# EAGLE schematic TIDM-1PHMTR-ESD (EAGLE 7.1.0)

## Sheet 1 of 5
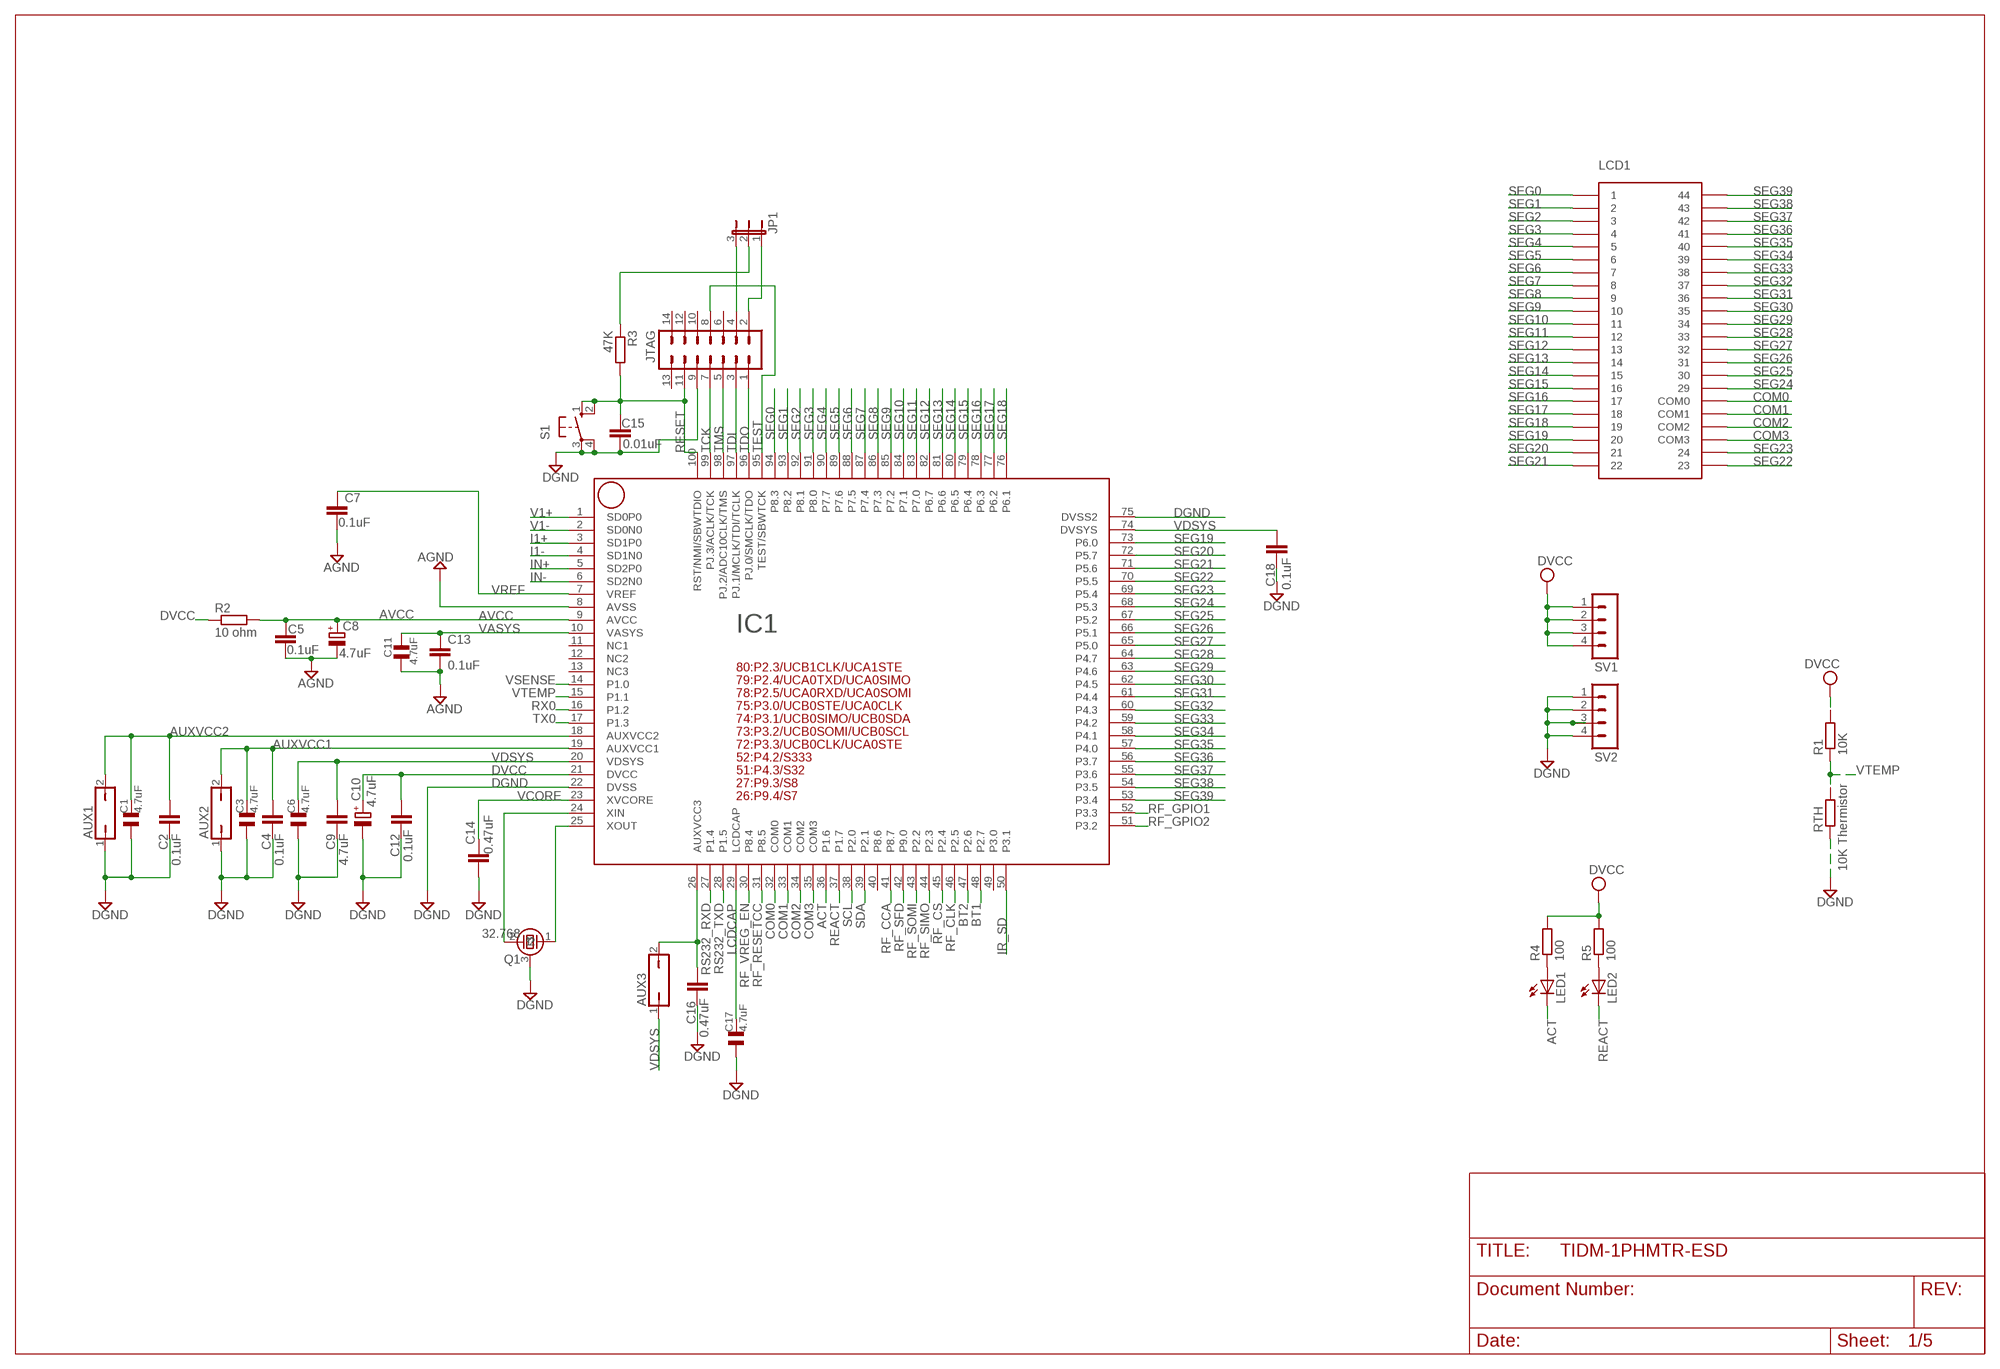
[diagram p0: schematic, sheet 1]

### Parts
AUX1  JP1Q  [JP1]
AUX2  JP1Q  [JP1]
AUX3  JP1Q  [JP1]
C1  4.7uF  C_0805  [0805]
C2  0.1uF  C-EUC0603  [C0603]
C3  4.7uF  C_0805  [0805]
C4  0.1uF  C-EUC0603  [C0603]
C5  0.1uF  C-EUC0603  [C0603]
C6  4.7uF  C_0805  [0805]
C7  0.1uF  C-EUC0603  [C0603]
C8  4.7uF  CPOL-EUSMCB  [SMC_B]
C9  4.7uF  C-EUC0603  [C0603]
C10  4.7uF  CPOL-EUSMCB  [SMC_B]
C11  4.7uF  C_0805  [0805]
C12  0.1uF  C-EUC0603  [C0603]
C13  0.1uF  C-EUC0603  [C0603]
C14  0.47uF  C-EUC0603  [C0603]
C15  0.01uF  C-EUC0603  [C0603]
C16  0.47uF  C-EUC0603  [C0603]
C17  4.7uF  C_0805  [0805]
C18  0.1uF  C-EUC0603  [C0603]
IC1  F6733---PZ100  [PZ100]
JP1  JP2E  [JP2]
JTAG  MA07-2MA07-2JTAG  [MA07-2JTAG]
LCD1  TI_160SEG_LCD  [TI_160SEG_LCD]
LED1  LED3MM  [LED3MM]
LED2  LED3MM  [LED3MM]
Q1  32.768  CRYSTAL-LSDTC26H-1  [TC26H-1]
R1  10K  R-EU_R0603  [R0603]
R2  10 ohm  R-EU_R0603  [R0603]
R3  47K  R-EU_R0603  [R0603]
R4  100  R-EU_R0603  [R0603]
R5  100  R-EU_R0603  [R0603]
RTH  10K Thermistor  R-EU_R0603  [R0603]
S1  10-XX  [B3F-10XX]
SV1  MA04-1  [MA04-1]
SV2  MA04-1  [MA04-1]

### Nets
ACT: IC1.36(P1.6) LED1.K(C) ; also sheet 4
AGND: C5.2 C7.2 C8.- C11.1 C13.2 IC1.8(AVSS) ; also sheet 2
AUXVCC1: AUX2.2 C3.2 C4.2 IC1.19(AUXVCC1)
AUXVCC2: AUX1.2 C1.2 C2.2 IC1.18(AUXVCC2)
AVCC: C5.1 C8.+ IC1.9(AVCC) R2.2 ; also sheet 2
BT1: IC1.48(P2.7) ; also sheet 4
BT2: IC1.47(P2.6) ; also sheet 4
COM0: IC1.32(COM0) LCD1.COM0
COM1: IC1.33(COM1) LCD1.COM1
COM2: IC1.34(COM2) LCD1.COM2
COM3: IC1.35(COM3) LCD1.COM3
DGND: AUX1.1 AUX2.1 C1.1 C2.1 C3.1 C4.1 C6.1 C9.1 C10.- C12.1 C14.1 C15.2 C16.1 C17.1 C18.1 IC1.22(DVSS) IC1.75(DVSS2) JTAG.9 Q1.3 RTH.1 S1.3(P) S1.4(P1) SV2.1 SV2.2 SV2.3 SV2.4 ; also sheet 3,4,5
DVCC: C10.+ C12.2 IC1.21(DVCC) JP1.2 R1.2 R2.1 R3.1 R4.2 R5.2 SV1.1 SV1.2 SV1.3 SV1.4 ; also sheet 3,4,5
I1+: IC1.3(SD1P0) ; also sheet 2
I1-: IC1.4(SD1N0) ; also sheet 2
IN+: IC1.5(SD2P0) ; also sheet 2
IN-: IC1.6(SD2N0) ; also sheet 2
IR_SD: IC1.50(P3.1) ; also sheet 4
JTAG_EXT: JP1.3 JTAG.4
JTAG_INT: JP1.1 JTAG.2
LCDCAP: C17.2 IC1.29(LCDCAP)
N$38: AUX3.2 C16.2 IC1.26(AUXVCC3)
N$104: LED1.A R4.1
N$105: LED2.A R5.1
REACT: IC1.37(P1.7) LED2.K(C) ; also sheet 4
RESET: C15.1 IC1.100(RST/NMI/SBWTDIO) JTAG.11 R3.2 S1.1(S) S1.2(S1)
RF_CCA: IC1.41(P8.7) ; also sheet 4
RF_CLK: IC1.46(P2.5) ; also sheet 4
RF_CS: IC1.45(P2.4) ; also sheet 4
RF_GPIO1: IC1.52(P3.3) ; also sheet 4
RF_GPIO2: IC1.51(P3.2) ; also sheet 4
RF_RESETCC: IC1.31(P8.5) ; also sheet 4
RF_SFD: IC1.42(P9.0) ; also sheet 4
RF_SIMO: IC1.44(P2.3) ; also sheet 4
RF_SOMI: IC1.43(P2.2) ; also sheet 4
RF_VREG_EN: IC1.30(P8.4) ; also sheet 4
RS232_RXD: IC1.27(P1.4) ; also sheet 5
RS232_TXD: IC1.28(P1.5) ; also sheet 5
RX0: IC1.16(P1.2) ; also sheet 4
SCL: IC1.38(P2.0) ; also sheet 4
SDA: IC1.39(P2.1) ; also sheet 4
SEG0: IC1.94(P8.3) LCD1.1
SEG1: IC1.93(P8.2) LCD1.2
SEG2: IC1.92(P8.1) LCD1.3
SEG3: IC1.91(P8.0) LCD1.4
SEG4: IC1.90(P7.7) LCD1.5
SEG5: IC1.89(P7.6) LCD1.6
SEG6: IC1.88(P7.5) LCD1.7
SEG7: IC1.87(P7.4) LCD1.8
SEG8: IC1.86(P7.3) LCD1.9
SEG9: IC1.85(P7.2) LCD1.10
SEG10: IC1.84(P7.1) LCD1.11
SEG11: IC1.83(P7.0) LCD1.12
SEG12: IC1.82(P6.7) LCD1.13
SEG13: IC1.81(P6.6) LCD1.14
SEG14: IC1.80(P6.5) LCD1.15
SEG15: IC1.79(P6.4) LCD1.16
SEG16: IC1.78(P6.3) LCD1.17
SEG17: IC1.77(P6.2) LCD1.18
SEG18: IC1.76(P6.1) LCD1.19
SEG19: IC1.73(P6.0) LCD1.20
SEG20: IC1.72(P5.7) LCD1.21
SEG21: IC1.71(P5.6) LCD1.22
SEG22: IC1.70(P5.5) LCD1.23
SEG23: IC1.69(P5.4) LCD1.24
SEG24: IC1.68(P5.3) LCD1.29
SEG25: IC1.67(P5.2) LCD1.30
SEG26: IC1.66(P5.1) LCD1.31
SEG27: IC1.65(P5.0) LCD1.32
SEG28: IC1.64(P4.7) LCD1.33
SEG29: IC1.63(P4.6) LCD1.34
SEG30: IC1.62(P4.5) LCD1.35
SEG31: IC1.61(P4.4) LCD1.36
SEG32: IC1.60(P4.3) LCD1.37
SEG33: IC1.59(P4.2) LCD1.38
SEG34: IC1.58(P4.1) LCD1.39
SEG35: IC1.57(P4.0) LCD1.40
SEG36: IC1.56(P3.7) LCD1.41
SEG37: IC1.55(P3.6) LCD1.42
SEG38: IC1.54(P3.5) LCD1.43
SEG39: IC1.53(P3.4) LCD1.44
TCK: IC1.99(PJ.3/ACLK/TCK) JTAG.7
TDI: IC1.97(PJ.1/MCLK/TDI/TCLK) JTAG.3
TDO: IC1.96(PJ.0/SMCLK/TDO) JTAG.1
TEST: IC1.95(TEST/SBWTCK) JTAG.8
TMS: IC1.98(PJ.2/ADC10CLK/TMS) JTAG.5
TX0: IC1.17(P1.3) ; also sheet 4
V1+: IC1.1(SD0P0) ; also sheet 2
V1-: IC1.2(SD0N0) ; also sheet 2
VASYS: C11.2 C13.1 IC1.10(VASYS)
VCORE: C14.2 IC1.23(XVCORE)
VDSYS: AUX3.1 C6.2 C9.2 C18.2 IC1.20(VDSYS) IC1.74(DVSYS)
VREF: C7.1 IC1.7(VREF)
VSENSE: IC1.14(P1.0) ; also sheet 3
VTEMP: IC1.15(P1.1) R1.1 RTH.2
XIN1: IC1.24(XIN) Q1.2
XOUT1: IC1.25(XOUT) Q1.1
Unconnected: IC1.11(NC1) IC1.12(NC2) IC1.13(NC3) IC1.40(P8.6) IC1.49(P3.0) JTAG.6 JTAG.10 JTAG.12 JTAG.13 JTAG.14

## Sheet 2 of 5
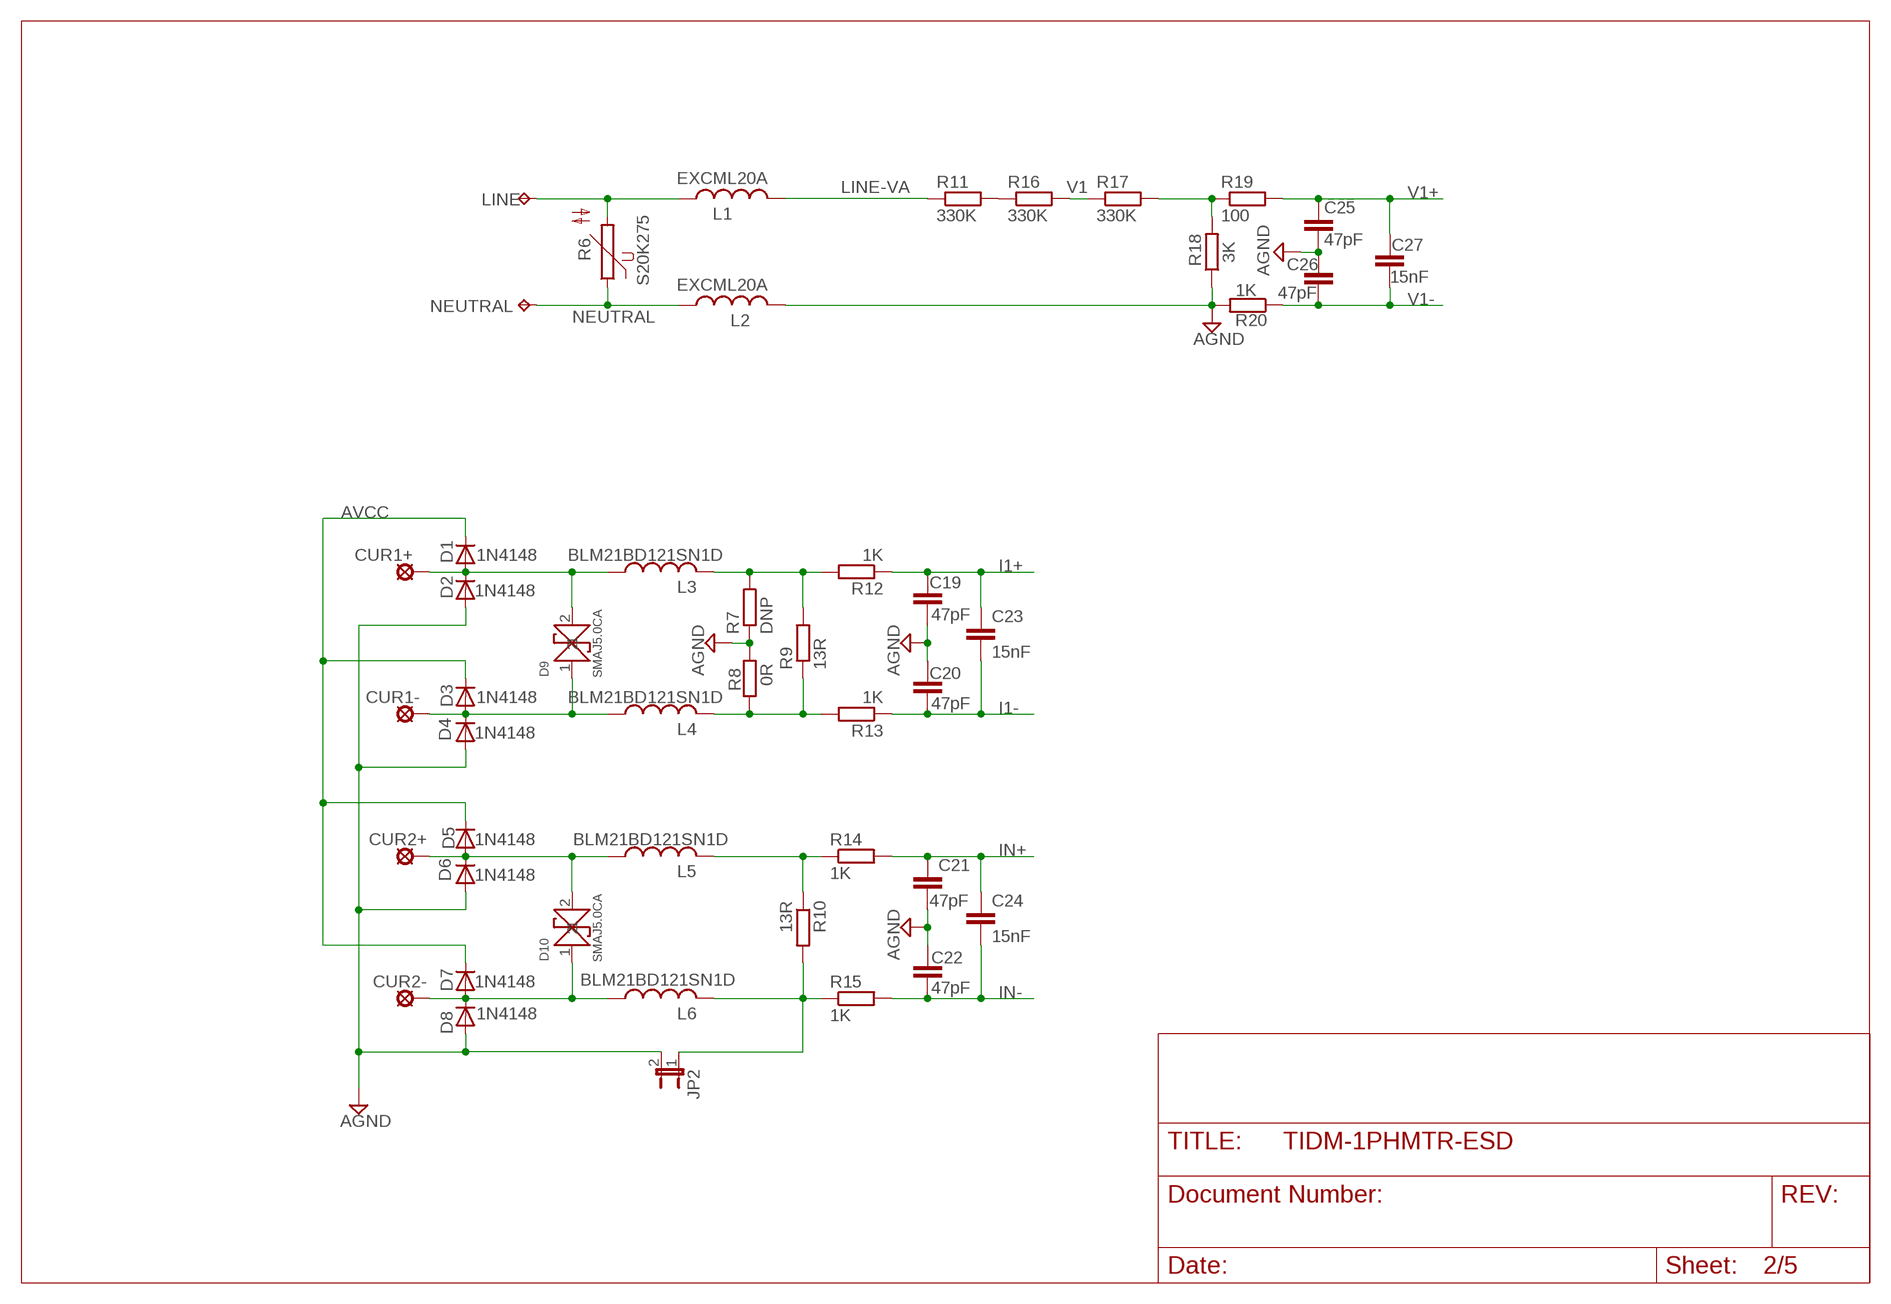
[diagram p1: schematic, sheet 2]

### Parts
C19  47pF  C-EUC0603  [C0603]
C20  47pF  C-EUC0603  [C0603]
C21  47pF  C-EUC0603  [C0603]
C22  47pF  C-EUC0603  [C0603]
C23  15nF  C-EUC0603  [C0603]
C24  15nF  C-EUC0603  [C0603]
C25  47pF  C-EUC0603  [C0603]
C26  47pF  C-EUC0603  [C0603]
C27  15nF  C-EUC0603  [C0603]
CUR1+  LSP10  [LSP10]
CUR1-  LSP10  [LSP10]
CUR2+  LSP10  [LSP10]
CUR2-  LSP10  [LSP10]
D1  1N4148  1N4148SOD80C  [SOD80C]
D2  1N4148  1N4148SOD80C  [SOD80C]
D3  1N4148  1N4148SOD80C  [SOD80C]
D4  1N4148  1N4148SOD80C  [SOD80C]
D5  1N4148  1N4148SOD80C  [SOD80C]
D6  1N4148  1N4148SOD80C  [SOD80C]
D7  1N4148  1N4148SOD80C  [SOD80C]
D8  1N4148  1N4148SOD80C  [SOD80C]
D9  SMAJ5.0CA  SMAJ  [DO-214]
D10  SMAJ5.0CA  SMAJ  [DO-214]
JP2  JP1E  [JP1]
L1  EXCML20A  L-US08050805  [0805@1]
L2  EXCML20A  L-US08050805  [0805@1]
L3  BLM21BD121SN1D  L-USL2012C  [L2012C]
L4  BLM21BD121SN1D  L-USL2012C  [L2012C]
L5  BLM21BD121SN1D  L-USL2012C  [L2012C]
L6  BLM21BD121SN1D  L-USL2012C  [L2012C]
LINE  TPPAD1-20  [P1-20]
NEUTRAL  TPPAD1-20  [P1-20]
R6  S20K275  S20K680S20K680-1  [S20K680-1]
R7  DNP  R-EU_R0603  [R0603]
R8  0R  R-EU_R0603  [R0603]
R9  13R  R-EU_R0603  [R0603]
R10  13R  R-EU_R0603  [R0603]
R11  330K  R-EU_R0603  [R0603]
R12  1K  R-EU_R0603  [R0603]
R13  1K  R-EU_R0603  [R0603]
R14  1K  R-EU_R0603  [R0603]
R15  1K  R-EU_R0603  [R0603]
R16  330K  R-EU_R0603  [R0603]
R17  330K  R-EU_R0603  [R0603]
R18  3K  R-EU_R0603  [R0603]
R19  100  R-EU_R0603  [R0603]
R20  1K  R-EU_R0603  [R0603]

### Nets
AGND: C19.2 C20.1 C21.2 C22.1 C25.2 C26.1 D2.A D4.A D6.A D8.A JP2.2 L2.2 R7.1 R8.2 R18.1 R20.2 ; also sheet 1
AVCC: D1.C D3.C D5.C D7.C ; also sheet 1
I1+: C19.1 C23.1 R12.1 ; also sheet 1
I1-: C20.2 C23.2 R13.1 ; also sheet 1
IN+: C21.1 C24.1 R14.2 ; also sheet 1
IN-: C22.2 C24.2 R15.2 ; also sheet 1
LINE-VA: L1.2 R11.1 ; also sheet 3
N$5: L1.1 LINE.TP R6.2
N$19: CUR1+.MP D1.A D2.C D9.2 L3.1
N$20: CUR1-.MP D3.A D4.C D9.1 L4.1
N$21: CUR2+.MP D5.A D6.C D10.2 L5.1
N$22: CUR2-.MP D7.A D8.C D10.1 L6.1
N$24: JP2.1 L6.2 R10.2 R15.1
N$27: L4.2 R8.1 R9.1 R13.2
N$31: L5.2 R10.1 R14.1
N$32: R17.2 R18.2 R19.1
N$39: R11.2 R16.1
N$42: L3.2 R7.2 R9.2 R12.2
NEUTRAL: L2.1 NEUTRAL.TP R6.1 ; also sheet 3
V1: R16.2 R17.1
V1+: C25.1 C27.1 R19.2 ; also sheet 1
V1-: C26.2 C27.2 R20.1 ; also sheet 1

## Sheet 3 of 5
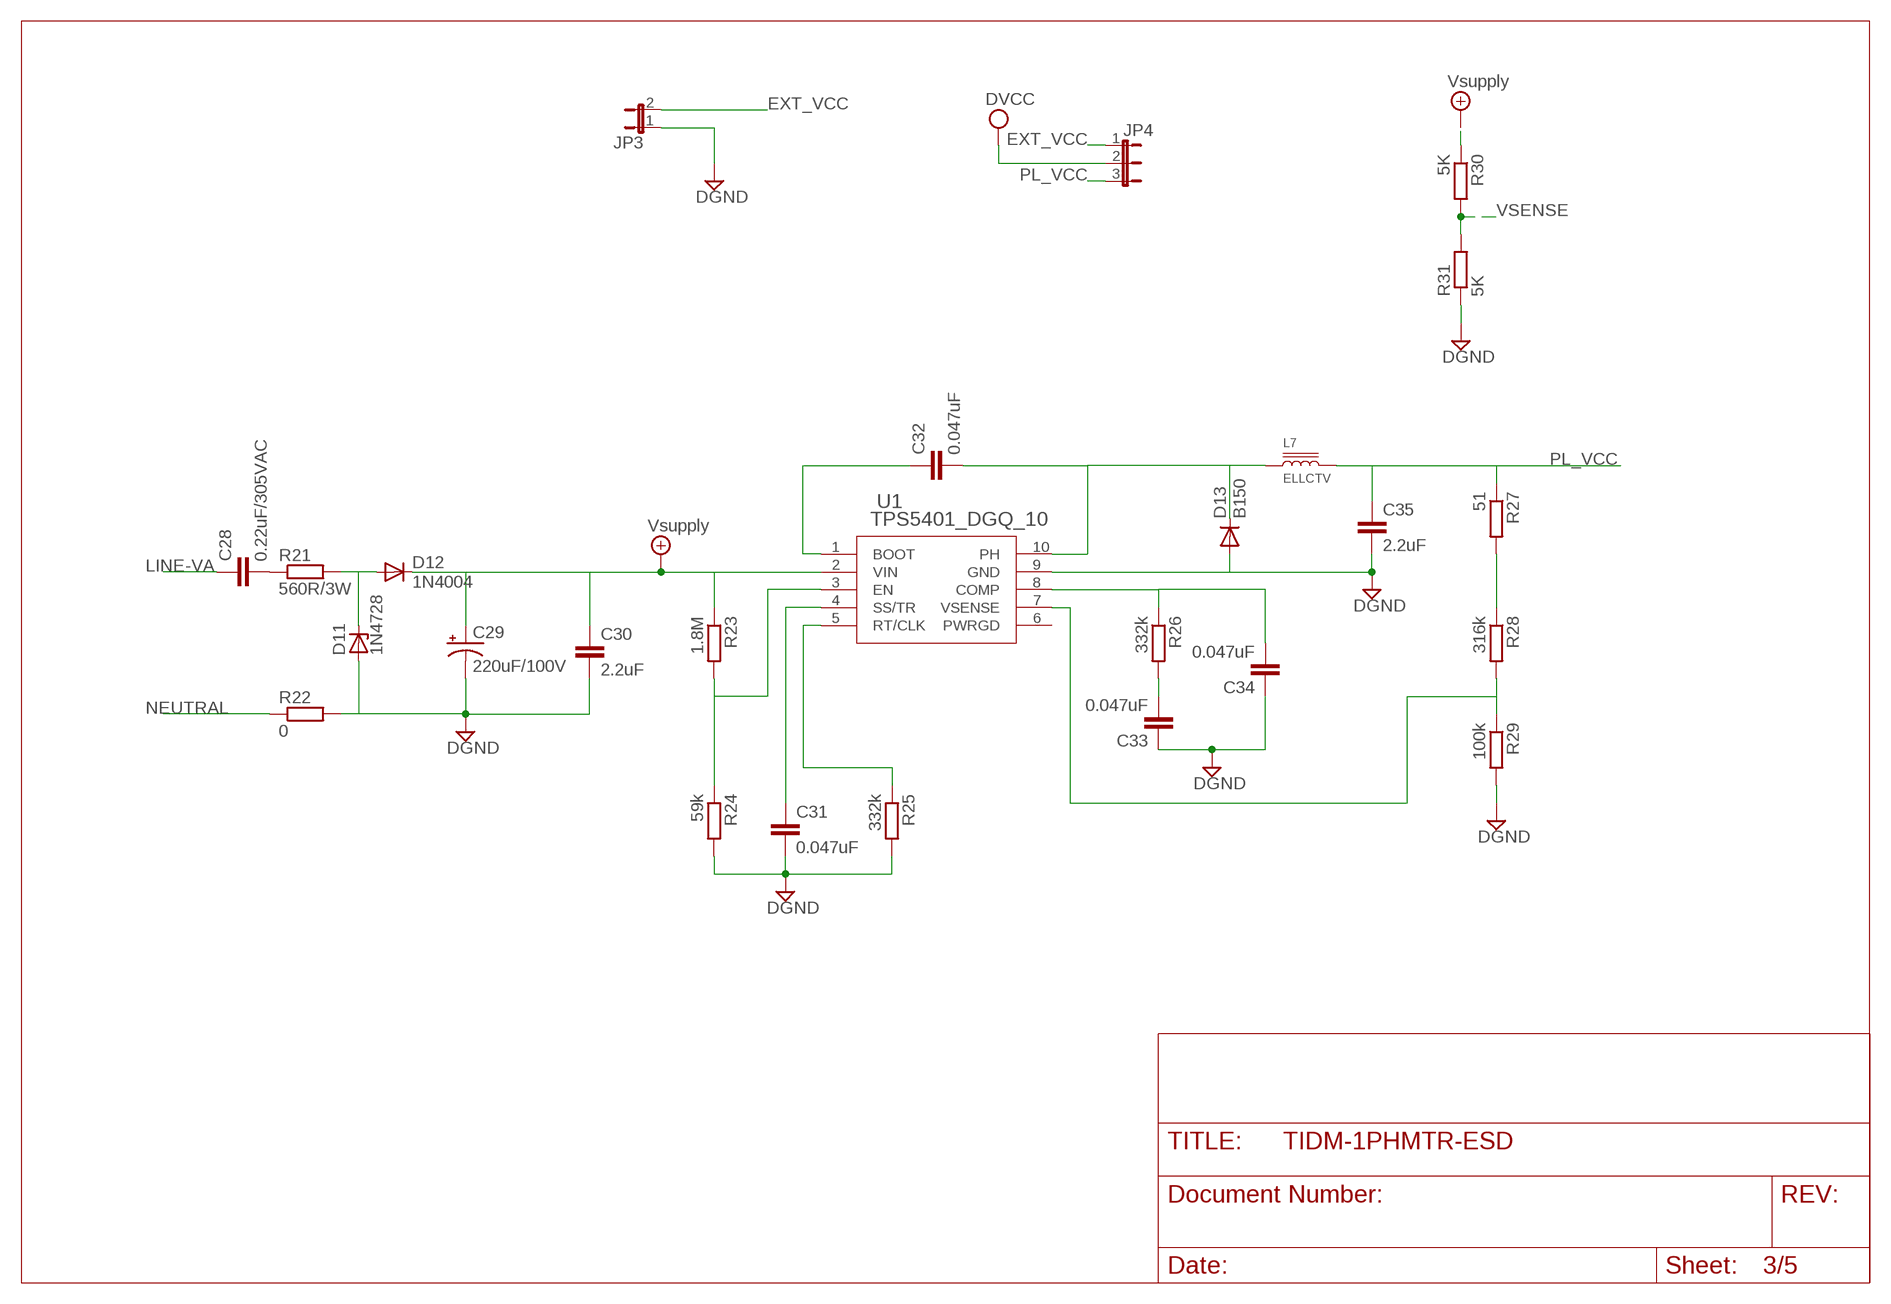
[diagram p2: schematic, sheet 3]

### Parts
C28  0.22uF/305VAC  C15/8  [C15B8]
C29  220uF/100V  CPOL-USE5-13  [E5-13]
C30  2.2uF  C-EUC1206  [C1206]
C31  0.047uF  C-EUC0603  [C0603]
C32  0.047uF  C-EUC0603  [C0603]
C33  0.047uF  C-EUC0603  [C0603]
C34  0.047uF  C-EUC0603  [C0603]
C35  2.2uF  C-EUC1206  [C1206]
D11  1N4728  [DO41Z10]
D12  1N4004  [DO41-10]
D13  B150  DIODE-DO214BA  [DO214BA]
JP3  JP1E  [JP1]
JP4  JP2E  [JP2]
L7  ELLCTV  [ELLCTV]
R21  560R/3W  R-EU_0414/15  [0414/15]
R22  0  R-EU_R0805  [R0805]
R23  1.8M  R-EU_R0603  [R0603]
R24  59k  R-EU_R0603  [R0603]
R25  332k  R-EU_R0603  [R0603]
R26  332k  R-EU_R0603  [R0603]
R27  51  R-EU_R0603  [R0603]
R28  316k  R-EU_R0603  [R0603]
R29  100k  R-EU_R0603  [R0603]
R30  5K  R-EU_R0603  [R0603]
R31  5K  R-EU_R0603  [R0603]
U1  TPS5401_DGQ_10  [DGQ10_1P88X1P57]

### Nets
+9V: C29.+ C30.1 D12.C R23.1 R30.1 U1.2(VIN) ; supply symbol labelled Vsupply
DGND: C29.- C30.2 C31.2 C33.1 C34.1 C35.2 D11.A D13.A JP3.1 R22.2 R24.2 R25.2 R29.2 R31.1 U1.9(GND) ; also sheet 1,4,5
DVCC: JP4.2 ; also sheet 1,4,5
EXT_VCC: JP3.2 JP4.1
LINE-VA: C28.1 ; also sheet 2
N$1: C28.2 R21.1
N$3: D11.C D12.A R21.2
N$7: R23.2 R24.1 U1.3(EN)
N$12: C31.1 U1.4(SS/TR)
N$13: R25.1 U1.5(RT/CLK)
N$23: C33.2 R26.2
N$25: R27.2 R28.1
N$26: C34.2 R26.1 U1.8(COMP)
N$28: C32.1 U1.1(BOOT)
N$29: C32.2 D13.C L7.1 U1.10(PH)
N$34: R28.2 R29.1 U1.7(VSENSE)
NEUTRAL: R22.1 ; also sheet 2
PL_VCC: C35.1 JP4.3 L7.2 R27.1
VSENSE: R30.2 R31.2 ; also sheet 1
Unconnected: U1.6(PWRGD)

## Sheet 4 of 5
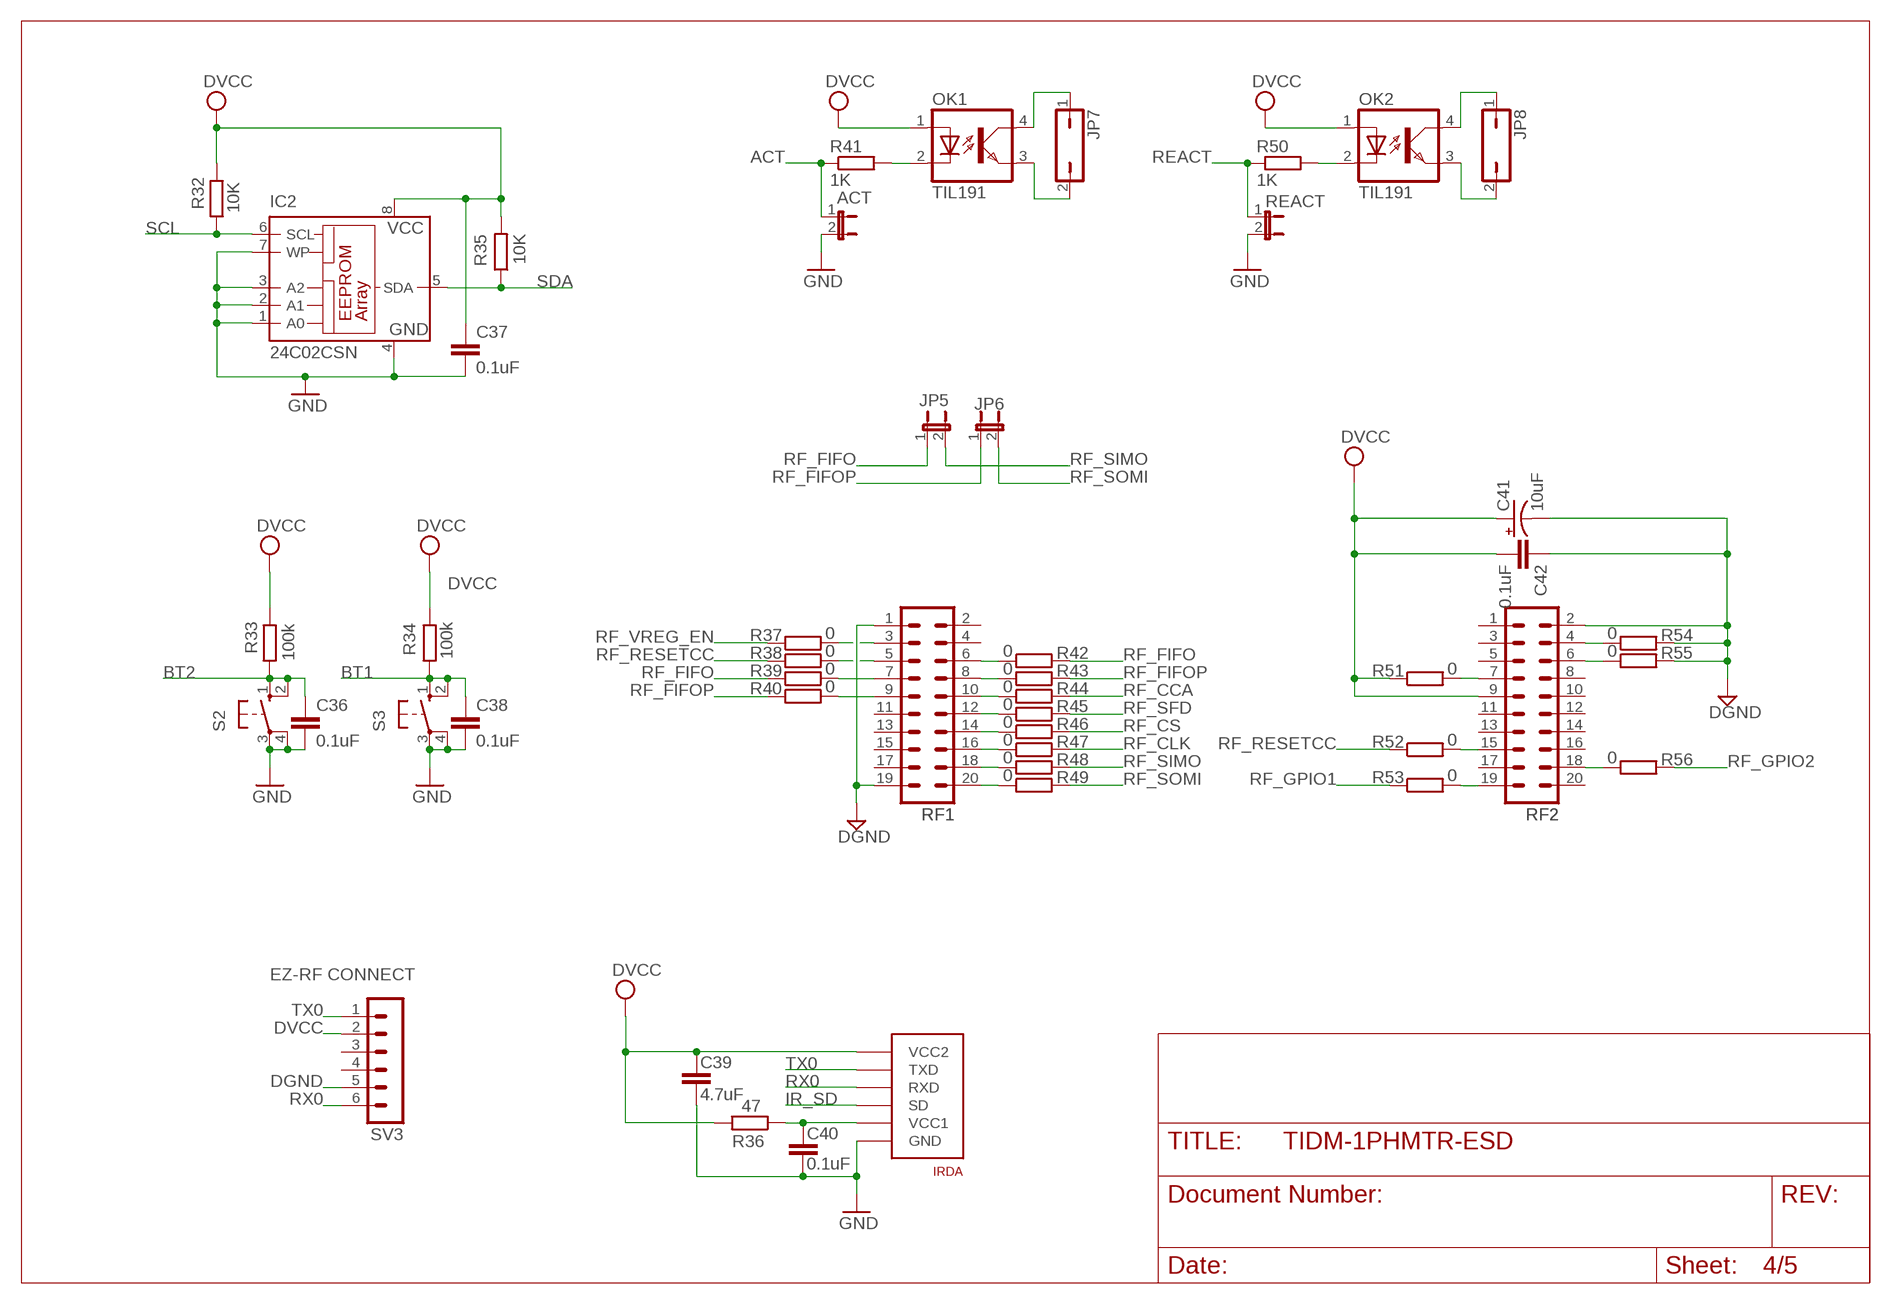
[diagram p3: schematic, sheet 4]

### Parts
ACT  JP1E  [JP1]
C36  0.1uF  C-EUC0603  [C0603]
C37  0.1uF  C-EUC0603  [C0603]
C38  0.1uF  C-EUC0603  [C0603]
C39  4.7uF  C-EUC0603  [C0603]
C40  0.1uF  C-EUC0603  [C0603]
C41  10uF  CPOL-USCT3216  [CT3216]
C42  0.1uF  C-EUC0603  [C0603]
IC2  24C02CSN  [SO-08]
IRDA  TFBS4711-TT1  [TFBS4711]
JP5  JP1E  [JP1]
JP6  JP1E  [JP1]
JP7  JP1Q  [JP1]
JP8  JP1Q  [JP1]
OK1  TIL191  [DIL04]
OK2  TIL191  [DIL04]
R32  10K  R-EU_R0603  [R0603]
R33  100k  R-EU_R0603  [R0603]
R34  100k  R-EU_R0603  [R0603]
R35  10K  R-EU_R0603  [R0603]
R36  47  R-EU_R0603  [R0603]
R37  0  R-EU_R0603  [R0603]
R38  0  R-EU_R0603  [R0603]
R39  0  R-EU_R0603  [R0603]
R40  0  R-EU_R0603  [R0603]
R41  1K  R-EU_R0603  [R0603]
R42  0  R-EU_R0603  [R0603]
R43  0  R-EU_R0603  [R0603]
R44  0  R-EU_R0603  [R0603]
R45  0  R-EU_R0603  [R0603]
R46  0  R-EU_R0603  [R0603]
R47  0  R-EU_R0603  [R0603]
R48  0  R-EU_R0603  [R0603]
R49  0  R-EU_R0603  [R0603]
R50  1K  R-EU_R0603  [R0603]
R51  0  R-EU_R0603  [R0603]
R52  0  R-EU_R0603  [R0603]
R53  0  R-EU_R0603  [R0603]
R54  0  R-EU_R0603  [R0603]
R55  0  R-EU_R0603  [R0603]
R56  0  R-EU_R0603  [R0603]
REACT  JP1E  [JP1]
RF1  TFM-110-02-SM-D-A-K  [TFM-110-02-SM-D-A-K]
RF2  TFM-110-02-SM-D-A-K  [TFM-110-02-SM-D-A-K]
S2  10-XX  [B3F-10XX]
S3  10-XX  [B3F-10XX]
SV3  MA06-1MA06-1-1.27  [MA06-1-1.27]

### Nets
ACT: ACT.1 R41.1 ; also sheet 1
BT1: C38.1 R34.1 S3.1(S) S3.2(S1) ; also sheet 1
BT2: C36.1 R33.1 S2.1(S) S2.2(S1) ; also sheet 1
DGND: ACT.2 C36.2 C37.2 C38.2 C39.2 C40.2 C41.- C42.1 IC2.1(A0) IC2.2(A1) IC2.3(A2) IC2.4(GND) IC2.7(WP) IRDA.P$6(GND) R54.2 R55.2 REACT.2 RF1.1 RF1.19 RF2.2 S2.3(P) S2.4(P1) S3.3(P) S3.4(P1) SV3.5 ; supply symbol labelled GND ; also sheet 1,3,5
DVCC: C37.1 C39.1 C41.+ C42.2 IC2.8(VCC) IRDA.P$1(VCC2) OK1.1(A) OK2.1(A) R32.2 R33.2 R34.2 R35.2 R36.2 R51.1 RF2.9 SV3.2 ; also sheet 1,3,5
IR_SD: IRDA.P$4(SD) ; also sheet 1
N$2: C40.1 IRDA.P$5(VCC1) R36.1
N$35: R37.2 RF1.3
N$45: R38.2 RF1.5
N$50: R51.2 RF2.7
N$51: R54.1 RF2.4
N$52: R52.2 RF2.15
N$53: R55.1 RF2.6
N$55: R44.1 RF1.10
N$56: R45.1 RF1.12
N$57: R46.1 RF1.14
N$59: R47.1 RF1.16
N$60: R48.1 RF1.18
N$61: R49.1 RF1.20
N$81: R53.2 RF2.19
N$83: R56.1 RF2.18
N$85: R39.2 RF1.7
N$86: R40.2 RF1.9
N$87: R43.1 RF1.8
N$88: R42.1 RF1.6
N$109: JP7.1 OK1.4(COL)
N$113: OK2.2(C) R50.2
N$114: OK1.2(C) R41.2
N$117: JP7.2 OK1.3(EMIT)
N$118: JP8.1 OK2.4(COL)
N$119: JP8.2 OK2.3(EMIT)
REACT: R50.1 REACT.1 ; also sheet 1
RF_CCA: R44.2 ; also sheet 1
RF_CLK: R47.2 ; also sheet 1
RF_CS: R46.2 ; also sheet 1
RF_FIFO: JP5.1 R39.1 R42.2
RF_FIFOP: JP6.1 R40.1 R43.2
RF_GPIO1: R53.1 ; also sheet 1
RF_GPIO2: R56.2 ; also sheet 1
RF_RESETCC: R38.1 R52.1 ; also sheet 1
RF_SFD: R45.2 ; also sheet 1
RF_SIMO: JP5.2 R48.2 ; also sheet 1
RF_SOMI: JP6.2 R49.2 ; also sheet 1
RF_VREG_EN: R37.1 ; also sheet 1
RX0: IRDA.P$3(RXD) SV3.6 ; also sheet 1
SCL: IC2.6(SCL) R32.1 ; also sheet 1
SDA: IC2.5(SDA) R35.1 ; also sheet 1
TX0: IRDA.P$2(TXD) SV3.1 ; also sheet 1
Unconnected: RF1.2 RF1.4 RF1.11 RF1.13 RF1.15 RF1.17 RF2.1 RF2.3 RF2.5 RF2.8 RF2.10 RF2.11 RF2.12 RF2.13 RF2.14 RF2.16 RF2.17 RF2.20 SV3.3 SV3.4

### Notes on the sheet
- EZ-RF CONNECT

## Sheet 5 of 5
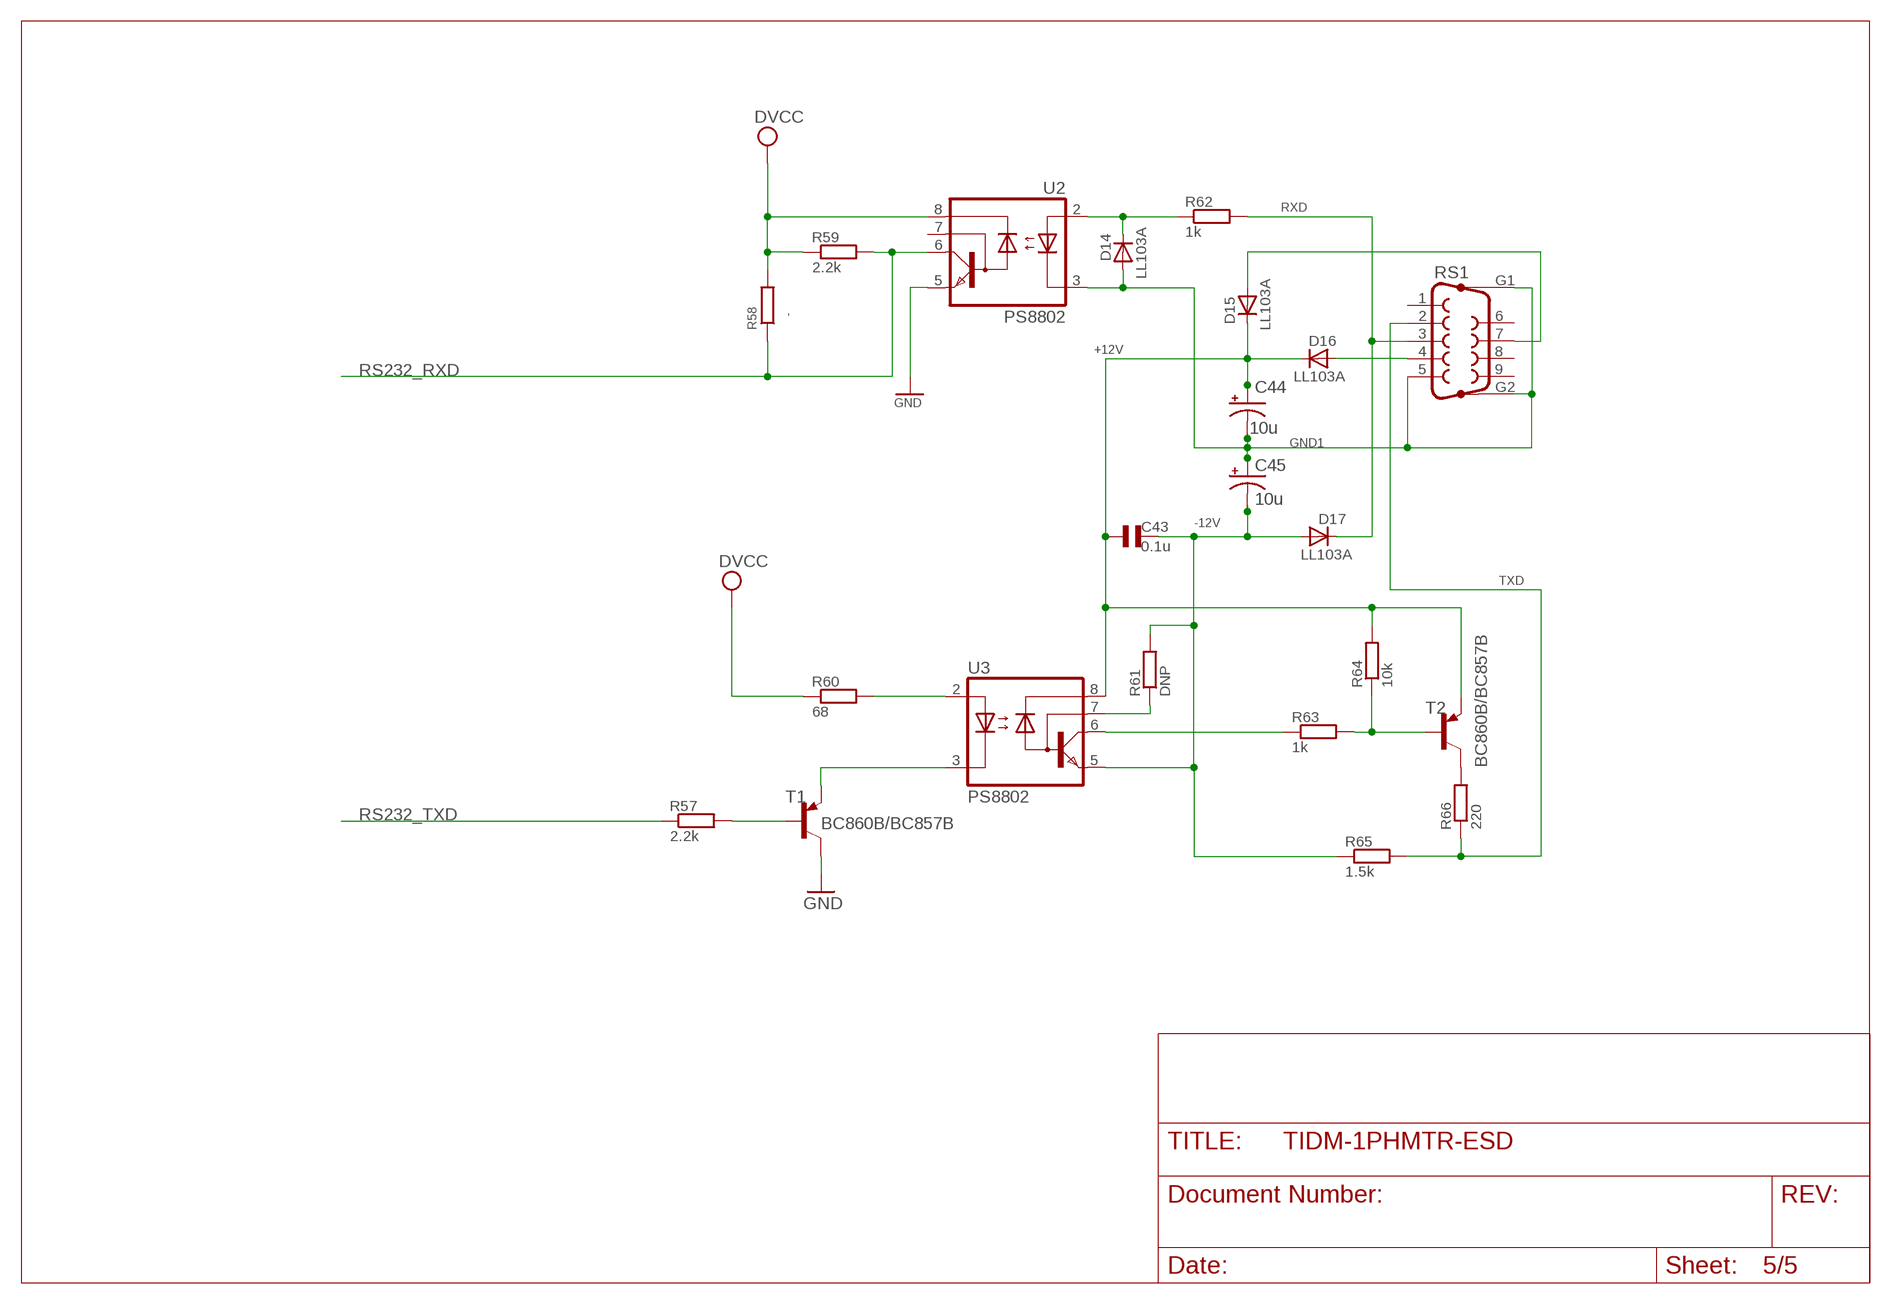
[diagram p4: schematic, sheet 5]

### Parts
C43  0.1u  CSMD0805  [CSMD0805]
C44  10u  CPOL-USCT3216  [CT3216]
C45  10u  CPOL-USCT3216  [CT3216]
D14  LL103A  D  [SOD-80]
D15  LL103A  D  [SOD-80]
D16  LL103A  D  [SOD-80]
D17  LL103A  D  [SOD-80]
R57  2.2k  R_0805  [0805]
R58  -  0204/5  [0805]
R59  2.2k  R_0805  [0805]
R60  68  R_0805  [0805]
R61  DNP  R_0805  [0805]
R62  1k  R_0805  [0805]
R63  1k  R_0805  [0805]
R64  10k  R_0805  [0805]
R65  1.5k  R_0805  [0805]
R66  220  R_0805  [0805]
RS1  F09VP  [F09VP]
T1  BC860B/BC857B  BC857ASMD  [SOT23-BEC]
T2  BC860B/BC857B  BC857ASMD  [SOT23-BEC]
U2  PS8802  PS8802SO08  [SO08]
U3  PS8802  PS8802SO08  [SO08]

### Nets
+12V: C43.1 C44.+ D15.2(K) D16.2(K) R64.2 T2.E U3.8(VCC)
+12V2: D15.1(A) RS1.7
+12V3: D16.1(A) RS1.4
-12V: C43.2 C45.- D17.1(A) R61.2 R65.1 U3.5(GND)
DGND: T1.C U2.5(GND) ; supply symbol labelled GND ; also sheet 1,3,4
DVCC: R58.2 R59.1 R60.1 U2.8(VCC) ; also sheet 1,3,4
GND1: C44.- C45.+ D14.1(A) RS1.5 RS1.G1 RS1.G2 U2.3(C)
N$14: D14.2(K) R62.1 U2.2(A)
N$15: R61.1 U3.7(VB)
N$16: R63.1 U3.6(VO)
N$17: R66.2 T2.C
N$18: R57.2 T1.B
N$30: R63.2 R64.1 T2.B
N$49: R60.2 U3.2(A)
N$455: T1.E U3.3(C)
RS232_RXD: R58.1 R59.2 U2.6(VO) ; also sheet 1
RS232_TXD: R57.1 ; also sheet 1
RXD: D17.2(K) R62.2 RS1.3
TXD: R65.2 R66.1 RS1.2
Unconnected: RS1.1 RS1.6 RS1.8 RS1.9 U2.7(VB)

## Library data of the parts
ACT JP2 JP3 JP5 JP6 REACT = custom_jumper:JP1E: JUMPER
AUX1-AUX3 JP7 JP8 = ElecMeter:JP1Q: JUMPER
C1 C3 C6 C11 C17 = ssmd:C_0805
C2 C4 C5 C7 C9 C12-C16 C18-C27 C31-C34 C36-C40 = ElecMeter:C-EU: CAPACITOR, European symbol
C8 C10 = ElecMeter:CPOL-EU: POLARIZED CAPACITOR, European symbol
C28 = capacitor-wima:C: CAPACITOR
C29 = resistor:CPOL-US: POLARIZED CAPACITOR, American symbol
C30 C35 = rcl:C-EU: CAPACITOR, European symbol
C41 C44 C45 = rcl:CPOL-US: POLARIZED CAPACITOR, American symbol
C42 = resistor:C-EU: CAPACITOR, European symbol
C43 = CAP:CSMD0805
CUR1+ CUR1- CUR2+ CUR2- = ElecMeter:LSP10: SOLDER PAD
D1-D8 = ElecMeter:1N4148: DIODE
D9 D10 = CON1:SMAJ
D11 = diode:1N4728: Z DIODE
D12 = diode:1N4004: DIODE
D13 = diode:DIODE-: DIODE
D14-D17 = SMD:D
IC1 = partslibTI_MSP430_v122:F6733---PZ100
IC2 = ElecMeter:24C*: Serial EEPROM 1 K/2 K/4 K
IRDA = Personal:TFBS4711-TT1
JP1 JP4 = custom_jumper:JP2E: JUMPER
JTAG = ElecMeter:MA07-2: PIN HEADER
L1 L2 = SMD:L-US0805
L3-L6 = ElecMeter:L-US: INDUCTOR, American symbol
L7 = ELLCTV:ELLCTV
LCD1 = Personal:TI_160SEG_LCD
LED1 LED2 = ElecMeter:LED: LED
LINE NEUTRAL = testpad:TP: Test pad
OK1 OK2 = ElecMeter:TIL191: TEXAS INSTRUMENTS OPTO COUPLER
Q1 = ElecMeter:CRYSTAL-LSD
R1-R5 R7-R20 R23-R36 R41 R50 RTH = ElecMeter:R-EU_: RESISTOR, European symbol
R6 = ElecMeter:S20K680: VARISTOR
R21 R37-R40 R42-R49 R51-R56 = rcl:R-EU_: RESISTOR, European symbol
R22 = resistors_with_outline:R-EU_: RESISTOR, European symbol
R57 R59-R66 = SMD:R_0805
R58 = R:0204/5
RF1 RF2 = _MSP430:TFM-110-02-SM-D-A-K
RS1 = con-subd:F09VP: SUB-D; OC_FARNELL: unknown; OC_NEWARK: unknown
S1-S3 = ElecMeter:10-XX: OMRON SWITCH
SV1 SV2 = custom_con-lstb:MA04-1: PIN HEADER; OC_FARNELL: unknown; OC_NEWARK: unknown
SV3 = con-lstb:MA06-1: PIN HEADER
T1 T2 = transistor-pnp:BC857*: PNP Transistror
U1 = TPS5401_DGQ_10:TPS5401_DGQ_10; DATASHEETURL: http://www.ti.com/lit/gpn/TPS5401; DESCRIPTION: 3.5V to 42V Input, 0.5 A Step Down Converter; FAMILY_NAME: STEP-DOWN REGULATOR; GENERIC_PART_NUMBER: TPS5401; INDUSTRY_STD_PKG_TYPE: MSOP-PowerPAD; MANUFACTURER: Texas Instruments; MANUFACTURER_PART_NUMBER: tps5401_dgq_10; PACKAGE_DESIGNATOR: DGQ; PIN_COUNT: 10; VENDOR: Texas Instruments
U2 U3 = FE449x EVM:PS8802: MOTOROLA OPTO COUPLER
